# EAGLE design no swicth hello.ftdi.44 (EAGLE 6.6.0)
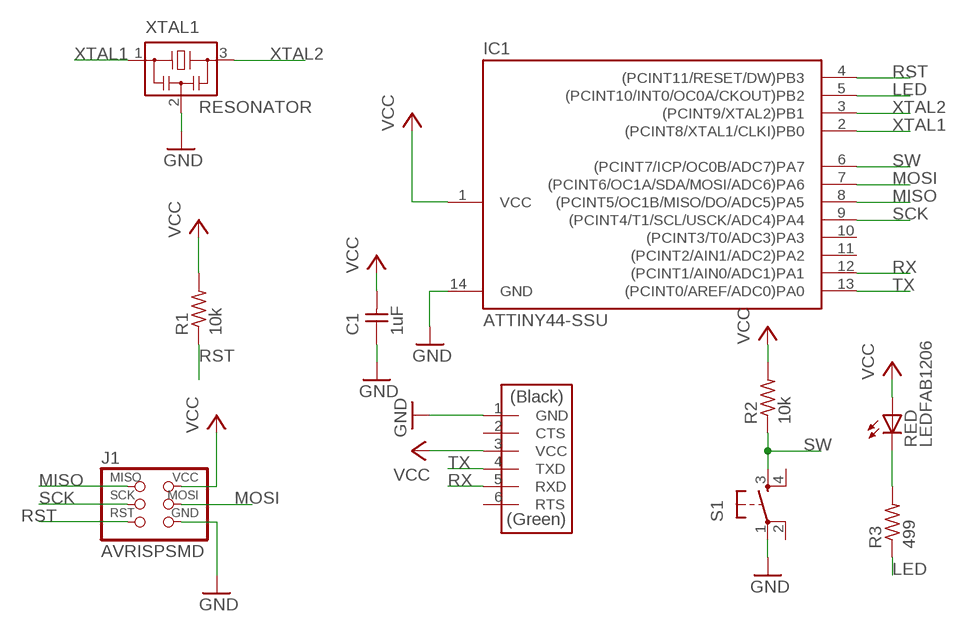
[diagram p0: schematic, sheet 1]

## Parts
C1  1uF  CAP-UNPOLARIZEDFAB  [C1206FAB]
IC1  ATTINY44-SSU  [SOIC14]
J1  AVRISPSMD  [2X03SMD]
J2  FTDI-SMD-HEADER  [1X06SMD]
R1  10k  RES-US1206FAB  [R1206FAB]
R2  10k  RES-US1206FAB  [R1206FAB]
R3  499  RES-US1206FAB  [R1206FAB]
RED  LEDFAB1206  [LED1206FAB]
S1  6MM_SWITCH6MM_SWITCH  [6MM_SWITCH]
XTAL1  RESONATOR  [EFOBM]

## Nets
GND: C1.1 IC1.14(GND) J1.6(GND) J2.1(GND) S1.1(P) XTAL1.2
LED: IC1.5((PCINT10/INT0/OC0A/CKOUT)PB2) R3.1
MISO: IC1.8((PCINT5/OC1B/MISO/DO/ADC5)PA5) J1.1(MISO)
MOSI: IC1.7((PCINT6/OC1A/SDA/MOSI/ADC6)PA6) J1.4(MOSI)
N$1: R3.2 RED.2(C)
RST: IC1.4((PCINT11/RESET/DW)PB3) J1.5(RST) R1.1
RX: IC1.12((PCINT1/AIN0/ADC1)PA1) J2.5(RXD)
SCK: IC1.9((PCINT4/T1/SCL/USCK/ADC4)PA4) J1.3(SCK)
SW: IC1.6((PCINT7/ICP/OC0B/ADC7)PA7) R2.1 S1.3(S)
TX: IC1.13((PCINT0/AREF/ADC0)PA0) J2.4(TXD)
VCC: C1.2 IC1.1(VCC) J1.2(VCC) J2.3(VCC) R1.2 R2.2 RED.1(A)
XTAL1: IC1.2((PCINT8/XTAL1/CLKI)PB0) XTAL1.1
XTAL2: IC1.3((PCINT9/XTAL2)PB1) XTAL1.3
Unconnected: IC1.10((PCINT3/T0/ADC3)PA3) IC1.11((PCINT2/AIN1/ADC2)PA2) J2.2(CTS) J2.6(RTS) S1.2(P1) S1.4(S1)

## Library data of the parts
C1 = fab:CAP-UNPOLARIZED
IC1 = fab:ATTINY44
J1 = fab:AVRISP
J2 = fab:FTDI-SMD-HEADER
R1-R3 = fab:RES-US: Resistor (US Symbol)
RED = fab:LED: LED
S1 = fab:6MM_SWITCH: OMRON SWITCH
XTAL1 = fab:RESONATOR

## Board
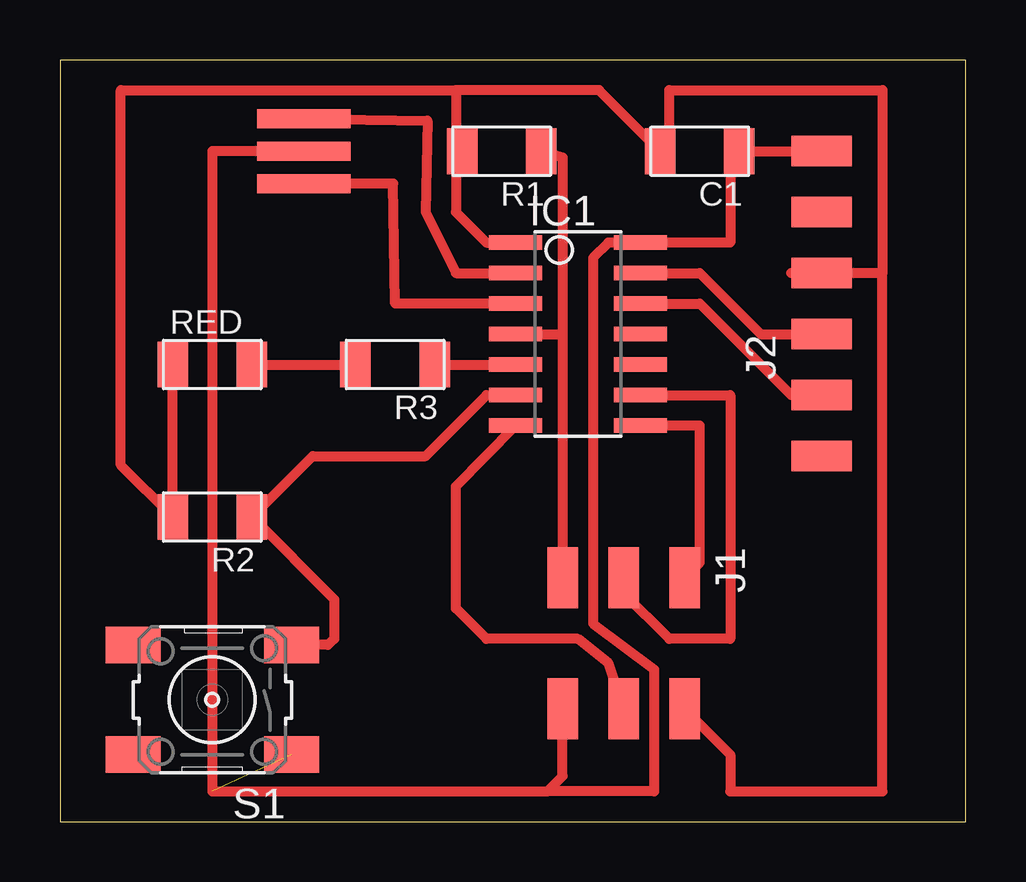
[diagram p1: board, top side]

Size 37.77 x 31.74 mm. Coordinates in mm from the lower left corner, seen from the top.
Outline: 0,0 37.77,0 37.77,31.74 0,31.74 0,0
Copper layers (1*16): Top 0.035mm / dielectric 1.5mm / Bottom 0.035mm
Design rules "fabmodule": minimum track width 10mil, minimum drill 0.4mm, track to track 0.42mm, track to pad 0.42mm, pad to pad 0.42mm, via to via 0.42mm, smd to smd 0.42mm, copper to edge 40mil, drill to drill 0.8mm, minimum pad ring 10mil, minimum via ring 8mil, stop-mask expansion 4mil, vias tented up to drill 0mil, thermal gap 10mil

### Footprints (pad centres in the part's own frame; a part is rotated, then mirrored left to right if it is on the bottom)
C1206FAB = smd 1.27 x 1.905: 1 -1.651,0; 2 1.651,0
SOIC14 = smd 0.61 x 2.21: 1 -3.81,-2.603; 2 -2.54,-2.603; 3 -1.27,-2.603; 4 0,-2.603; 5 1.27,-2.603; 6 2.54,-2.603; 7 3.81,-2.603; 8 3.81,2.603; 9 2.54,2.603; 10 1.27,2.603; 11 0,2.603; 12 -1.27,2.603; 13 -2.54,2.603; 14 -3.81,2.603
2X03SMD = smd 2.54 x 1.27: 1 -2.54,2.54; 2 2.92,2.54; 3 -2.54,0; 4 2.92,0; 5 -2.54,-2.54; 6 2.92,-2.54
1X06SMD = smd 2.54 x 1.27: 1 0,6.35; 2 0,3.81; 3 0,1.27; 4 0,-1.27; 5 0,-3.81; 6 0,-6.35
R1206FAB = smd 1.27 x 1.905: 1 -1.651,0; 2 1.651,0
LED1206FAB = smd 1.27 x 1.905: 1 -1.651,0; 2 1.651,0
6MM_SWITCH = smd 2.286 x 1.524: 1 -3.302,2.286; 2 3.302,2.286; 3 -3.302,-2.286; 4 3.302,-2.286
EFOBM = smd 0.8 x 3.9: 1 -1.35,0; 2 0,0; 3 1.35,0

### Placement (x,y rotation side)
C1  26.67,27.94 180 top
IC1  21.59,20.32 270 top
J1  23.49,7.62 270 top
J2  31.75,21.59 0 top
R1  18.41,27.94 180 top
R2  6.35,12.7 180 top
R3  13.97,19.05 180 top
RED  6.35,19.05 0 top
S1  6.35,5.08 180 top
XTAL1  10.16,27.94 270 top

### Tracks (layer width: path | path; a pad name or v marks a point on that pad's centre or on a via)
GND  (1 unrouted)
  Top 0.406: J2.1 C1.1 27.94,27.56 27.94,24.13 IC1.14 22.86,24.13 22.23,23.49 22.23,8.26 24.77,6.35 24.77,1.27 20.32,1.27 | XTAL1.2 6.35,27.94 6.35,1.27 20.32,1.27 | 20.32,1.27 20.95,1.91 J1.6
LED
  Top 0.406: R3.1 IC1.5
MISO
  Top 0.406: J1.1 26.67,10.79 26.67,16.51 IC1.8
MOSI
  Top 0.406: J1.4 22.86,6.61 21.59,7.62 17.78,7.62 16.51,8.89 16.51,13.97 IC1.7
N$1
  Top 0.406: RED.2 R3.2
RST
  Top 0.406: R1.1 20.95,27.69 20.95,20.32 | 20.95,20.32 J1.5 | IC1.4 20.95,20.32
RX
  Top 0.406: IC1.12 26.67,21.59 30.48,17.78 J2.5
SCK
  Top 0.406: IC1.9 27.94,17.78 27.94,7.62 25.4,7.62 23.49,9.53 J1.3
SW
  Top 0.406: IC1.6 17.78,17.78 15.24,15.24 10.54,15.24 R2.1 11.43,9.27 11.43,7.62 11.18,7.37 S1.3
TX
  Top 0.406: IC1.13 26.67,22.86 29.21,20.32 J2.4
VCC
  Top 0.406: IC1.1 17.78,24.13 16.51,25.4 16.51,27.69 R1.2 16.51,27.94 16.51,30.48 | J1.2 27.94,2.79 27.94,1.27 34.29,1.27 34.29,22.86 | 34.29,22.86 J2.3 30.48,22.86 | 34.29,22.86 34.29,30.48 25.4,30.48 25.4,28.32 C1.2 22.48,30.48 17.78,30.48 16.51,30.48 | RED.1 R2.2 2.54,14.86 2.54,30.48 16.51,30.48
XTAL1
  Top 0.406: XTAL1.1 15.32,29.21 15.24,25.4 16.51,22.86 IC1.2
XTAL2
  Top 0.406: IC1.3 13.97,21.59 13.89,26.59 XTAL1.3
